FUNCTION "SCHALING-3" : VOID
TITLE =Schaling
AUTHOR : MJO
FAMILY : GEMAAL
NAME : SCHALING
VERSION : 0.1


VAR_INPUT
  In : REAL ;   //Ingangswaarde
  X1 : REAL ;   //X-waarde punt 1
  Y1 : REAL ;   //Y-waarde punt 1
  X2 : REAL ;   //X-warde punt 2
  Y2 : REAL ;   //Y-waarde punt 2
  X3 : REAL ;   //X-waarde punt 3
  Y3 : REAL ;   //Y-waarde punt 3
  Percent0 : REAL ; //0% waarde
  Percent100 : REAL ;   //100% waarde
END_VAR
VAR_OUTPUT
  Uit : REAL ;  //Uitgangswaarde
  Percentage : REAL ;   //Uitgangswaarde in %
END_VAR
VAR_TEMP
  A : REAL ;    //Schalingsconstante A
  B : REAL ;    //Schalingsconstante B
  TmpReal : REAL ;
  XX1 : REAL ;
  YY1 : REAL ;
  XX2 : REAL ;
  YY2 : REAL ;
END_VAR
BEGIN
NETWORK
TITLE =
//De schaling kent twee hellingshoeken, afhankelijk van de x-waarde wordt de
//hellingshoek geselecteerd. Is de x-waarde kleiner als X2 dan wordt de eerste
//hellingshoek gneomen, en anders de tweede.
      L     #In;
      L     #X2;
      >=R   ;
      JC    P2; //selecteer tweede hellingshoek
      L     #X1; //eerste punt is (x1,y1)
      T     #XX1;
      L     #Y1;
      T     #YY1;
      L     #X2; //tweede punt is (x2,y2)
      T     #XX2;
      L     #Y2;
      T     #YY2;
      JU    END;
P2:   L     #X2; //eerste punt is (x2,y2)
      T     #XX1;
      L     #Y2;
      T     #YY1;
      L     #X3; //tweede punt is (x3,y3)
      T     #XX2;
      L     #Y3;
      T     #YY2;
END:  NOP   0;
NETWORK
TITLE =Bereken constante A
//Berekenen constante A: A = (Uit2 - Uit1) / (In2 - In1)
//
      L     #XX2;
      L     #XX1;
      -R    ; //Berekend (In2 - In1)
      T     #TmpReal; //Tijdelijke opslag resultaat
      L     #YY2;
      L     #YY1;
      -R    ; //Berekend (Uit2 - Uit1)
      L     #TmpReal; //Ophalen (Uit2 - Uit1)
      /R    ; //Berekend (In2 - In1)/(Uit2 - Uit1)
      T     #A;
NETWORK
TITLE =Bereken constante B
//Berekenen constante B: B = Uit1 - (A * In1)
//
      L     #A;
      L     #XX1;
      *R    ; //Berekend (A * In1)
      T     #TmpReal; //Tijdelijke opslag resultaat
      L     #YY1;
      L     #TmpReal;
      -R    ; //Berekend Uit1 - (A * In1)
      T     #B;
NETWORK
TITLE =Bepaal uitgangswaarde
//
//
      L     #In;
      L     #A;
      *R    ;
      L     #B;
      +R    ;
      T     #Uit;
NETWORK
TITLE =Bepaal percentage
//Voor bepaling van percentage geldt: Y1 ~ 0% en Y2 ~ 100%.
//Uitganspercentage wordt berekend volgens:
//       x % = (#Uit - Y1) * 100 / (Y2 - Y1)
      L     #Percent100;
      L     #Percent0;
      -R    ;
      T     #TmpReal;
      L     #Uit;
      L     #Percent0;
      -R    ;
      L     1.000000e+002;
      *R    ;
      L     #TmpReal;
      /R    ;
      T     #Percentage;
END_FUNCTION
